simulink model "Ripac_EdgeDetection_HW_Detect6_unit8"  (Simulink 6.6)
settings: Solver=FixedStepDiscrete  SolverMode=SingleTasking  StartTime=0.0  StopTime=row  RelTol=1e-3
PreLoadFcn:
  | [r,g,b]=Ripac_img_start('image.jpg');
  | 
  | col=r.signals.dimensions;
  | row=size(r.signals.values,1);
  | 
  | kernel = [-1 0 1; -2 0 2; -1 0 1];
  | gain_frac=0;
InitFcn:
  | %[r,g,b]=Ripac_img_start('image.jpg');
  | 
  | %col=r.signals.dimensions;
  | %row=size(r.signals.values,1);
  | 
  | %kernel = [-1 0 1; -2 0 2; -1 0 1];
  | 
  | gain_frac=0;
StopFcn:
  | obr_out=Ripac_img_stop(hrana,col);
  | obr=int16((double(obr_out)).^(1/2));
  | figure, image(obr); colormap('gray'), title('Final Edge Detected Image')
  | 
  | output_struct=hrana8;
  | obr2_out=reshape(output_struct.signals.values(1:end-1),col+2,prod(size(output_struct.signals.values(1:end-1)))/(col+2))';
  | obr2=int16(obr2_out.^(1/2));
  | figure,image(obr2); colormap('gray'), title('HW Edge Detected Image')
libraries: syndsplibv9 x42, simulink x8, dspbuff3 x1

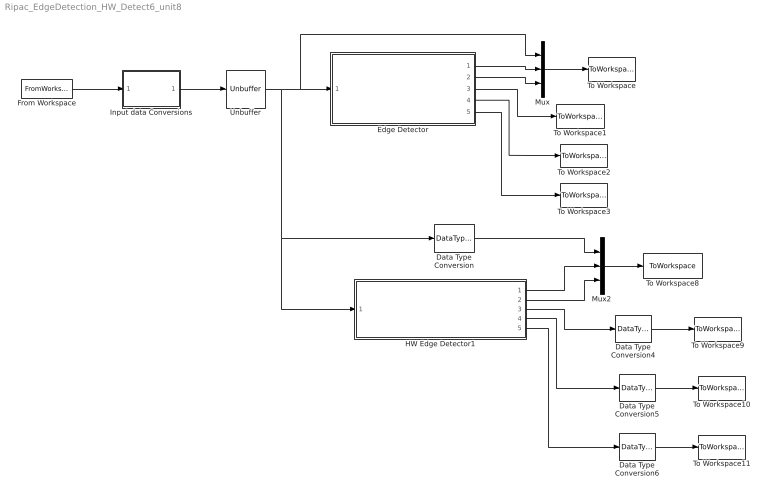
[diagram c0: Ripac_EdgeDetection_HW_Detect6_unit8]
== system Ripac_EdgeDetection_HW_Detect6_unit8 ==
  Data Type Conversion : DataTypeConversion  OutDataTypeMode=int16
  Data Type Conversion4 : DataTypeConversion  OutDataTypeMode=double  RndMeth=Nearest
  Data Type Conversion5 : DataTypeConversion  OutDataTypeMode=int32  RndMeth=Nearest
  Data Type Conversion6 : DataTypeConversion  OutDataTypeMode=int32  RndMeth=Nearest
  Edge Detector : Subsystem
  From Workspace : FromWorkspace  VariableName=r  SampleTime=0  Interpolate=off  OutputAfterFinalValue=Setting to zero
  HW Edge Detector1 : Subsystem
  Input data Conversions : Subsystem
  Mux : Mux  Inputs=3
  Mux2 : Mux  Inputs=3
  To Workspace : ToWorkspace  VariableName=simout  SampleTime=-1  SaveFormat=Structure With Time
  To Workspace1 : ToWorkspace  VariableName=hrana  SampleTime=-1  SaveFormat=Structure With Time
  To Workspace10 : ToWorkspace  VariableName=hrana6  SampleTime=-1  SaveFormat=Structure With Time
  To Workspace11 : ToWorkspace  VariableName=hrana7  SampleTime=-1  SaveFormat=Structure With Time
  To Workspace2 : ToWorkspace  VariableName=hrana1  SampleTime=-1  SaveFormat=Structure With Time
  To Workspace3 : ToWorkspace  VariableName=hrana2  SampleTime=-1  SaveFormat=Structure With Time
  To Workspace8 : ToWorkspace  VariableName=simout_HW1  SampleTime=-1  SaveFormat=Structure With Time
  To Workspace9 : ToWorkspace  VariableName=hrana8  SampleTime=-1  SaveFormat=Structure With Time
  Unbuffer : dspbuff3/Unbuffer  ic=0
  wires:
  From Workspace/1 -> Input data Conversions/1(In)
  Unbuffer/1 -> Mux/1, Edge Detector/1(Row Input), HW Edge Detector1/1(In1), Data Type Conversion/1
  Input data Conversions/1(Out) -> Unbuffer/1
  Edge Detector/3(Detector Out) -> To Workspace1/1
  Mux/1 -> To Workspace/1
  Edge Detector/1(Delay Line Out 1) -> Mux/2
  Edge Detector/2(Delay Line Out 2) -> Mux/3
  Edge Detector/4(Detector Out1) -> To Workspace2/1
  Edge Detector/5(Detector Out2) -> To Workspace3/1
  HW Edge Detector1/1(Delay Line 1) -> Mux2/2
  HW Edge Detector1/2("Delay Line 2 ") -> Mux2/3
  Mux2/1 -> To Workspace8/1
  Data Type Conversion4/1 -> To Workspace9/1
  Data Type Conversion5/1 -> To Workspace10/1
  HW Edge Detector1/3(Edge2) -> Data Type Conversion4/1
  HW Edge Detector1/4(Edge) -> Data Type Conversion5/1
  HW Edge Detector1/5(Edge1) -> Data Type Conversion6/1
  Data Type Conversion6/1 -> To Workspace11/1
  Data Type Conversion/1 -> Mux2/1

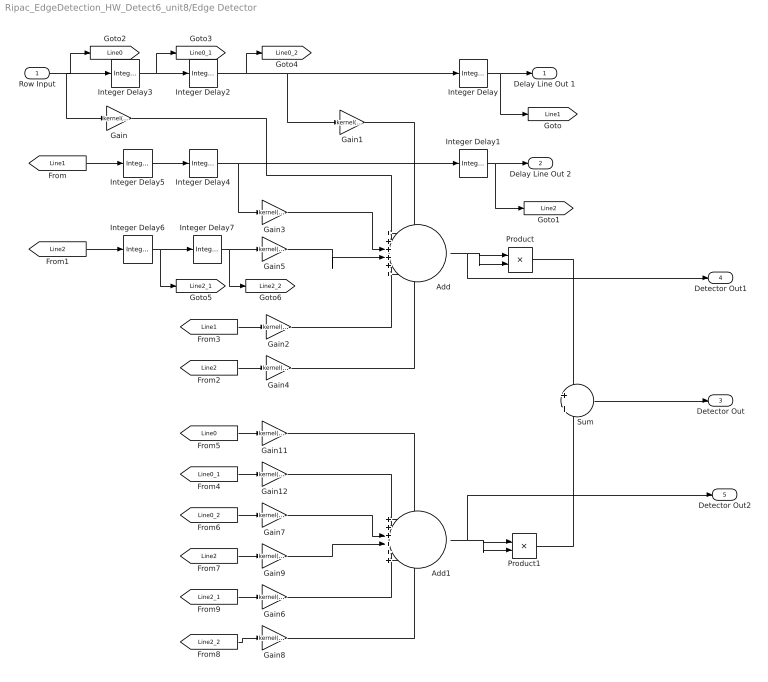
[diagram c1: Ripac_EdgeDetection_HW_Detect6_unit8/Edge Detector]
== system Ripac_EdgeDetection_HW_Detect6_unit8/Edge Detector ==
  Row Input : Inport  OutDataType=fixdt(1,16,0)  OutScaling=[]
  Add : Sum  Inputs=++++++  OutScaling=2^-10
  Add1 : Sum  Inputs=++++++  OutScaling=2^-10
  Gain : Gain  Gain=kernel(1,1)
  Gain1 : Gain  Gain=kernel(1,3)
  Gain11 : Gain  Gain=kernel(1,1)
  Gain12 : Gain  Gain=kernel(2,1)
  Gain2 : Gain  Gain=kernel(2,1)
  Gain3 : Gain  Gain=kernel(2,3)
  Gain4 : Gain  Gain=kernel(3,1)
  Gain5 : Gain  Gain=kernel(3,3)
  Gain6 : Gain  Gain=kernel(2,3)
  Gain7 : Gain  Gain=kernel(3,1)
  Gain8 : Gain  Gain=kernel(3,3)
  Gain9 : Gain  Gain=kernel(1,3)
  Integer Delay : simulink/Discrete/Integer Delay  vinit=0.0  samptime=-1  NumDelays=col
  Integer Delay1 : simulink/Discrete/Integer Delay  vinit=0.0  samptime=-1  NumDelays=col
  Integer Delay{2..7} (6 alike) : simulink/Discrete/Integer Delay  vinit=0.0  samptime=-1  NumDelays=1
  Product : Product  OutDataTypeMode=double
  Product1 : Product  OutDataTypeMode=double
  Sum : Sum  Inputs=+|+
  Delay Line Out 1 : Outport  OutDataType=fixdt(1,16,0)  OutScaling=[]
  Delay Line Out 2 : Outport  Port=2  OutDataType=fixdt(1,16,0)  OutScaling=[]
  Detector Out : Outport  Port=3  OutDataType=fixdt(1,16,0)  OutScaling=[]
  Detector Out1 : Outport  Port=4  OutDataType=fixdt(1,16,0)  OutScaling=[]
  Detector Out2 : Outport  Port=5  OutDataType=fixdt(1,16,0)  OutScaling=[]
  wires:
  Integer Delay/1 -> Delay Line Out 1/1, [Line1]
  Integer Delay3/1 -> [Line0_1], Integer Delay2/1
  Integer Delay2/1 -> Integer Delay/1, Gain1/1, [Line0_2]
  Integer Delay5/1 -> Integer Delay4/1
  Integer Delay4/1 -> Gain3/1, Integer Delay1/1
  Integer Delay6/1 -> [Line2_1], Integer Delay7/1
  Integer Delay7/1 -> Gain5/1, [Line2_2]
  Integer Delay1/1 -> Delay Line Out 2/1, [Line2]
  Gain1/1 -> Add/1
  Gain4/1 -> Add/6
  Row Input/1 -> Gain/1, [Line0], Integer Delay3/1
  [Line1] -> Integer Delay5/1
  [Line2] -> Integer Delay6/1
  [Line2] -> Gain4/1
  [Line1] -> Gain2/1
  Gain/1 -> Add/2
  Gain3/1 -> Add/3
  Gain5/1 -> Add/4
  Gain2/1 -> Add/5
  Gain11/1 -> Add1/1
  Gain8/1 -> Add1/6
  Add1/1 -> Product1/1, Product1/2, Detector Out2/1
  Gain12/1 -> Add1/2
  Gain7/1 -> Add1/3
  Gain9/1 -> Add1/4
  Gain6/1 -> Add1/5
  [Line0] -> Gain11/1
  [Line0_2] -> Gain7/1
  [Line0_1] -> Gain12/1
  [Line2] -> Gain9/1
  [Line2_1] -> Gain6/1
  [Line2_2] -> Gain8/1
  Add/1 -> Product/1, Product/2, Detector Out1/1
  Product/1 -> Sum/1
  Product1/1 -> Sum/2
  Sum/1 -> Detector Out/1

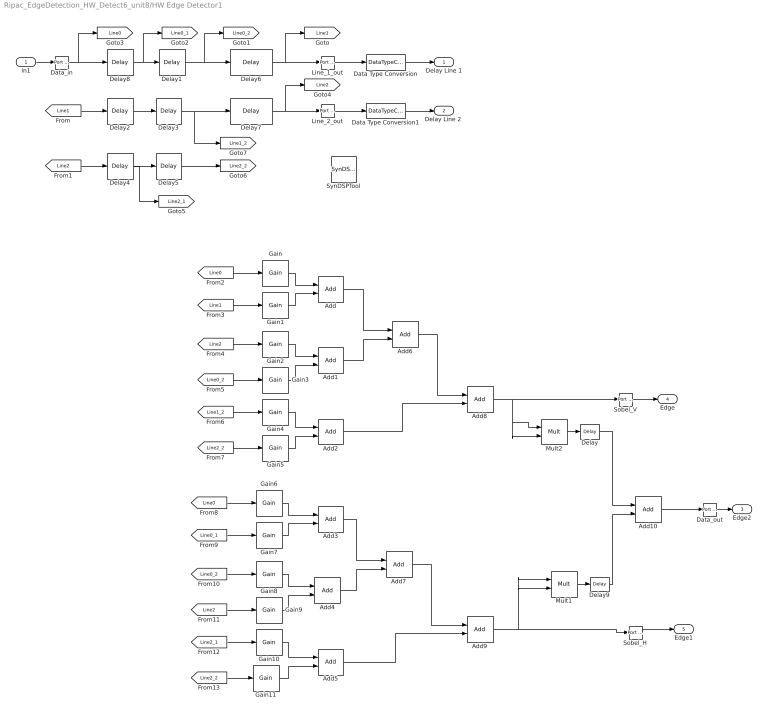
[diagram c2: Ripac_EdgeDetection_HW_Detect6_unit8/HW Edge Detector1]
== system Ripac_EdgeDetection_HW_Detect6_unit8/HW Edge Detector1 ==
  In1 : Inport  OutDataType=fixdt(1,16,0)  OutScaling=[]
  Add{,1..10} (11 alike) : syndsplibv9/Math Functions/Add  syn_add_opr=++  syn_out_f=Automatic  syn_out_wl=16  syn_out_fl=8  syn_out_dt=signed  syn_out_sat=off  syn_out_rnd=Floor (Truncate)  synBlockType=primitive  synLatency=0  synBlockId=96
  Data Type Conversion : DataTypeConversion  OutDataTypeMode=int16
  Data Type Conversion1 : DataTypeConversion  OutDataTypeMode=int16
  Data_in : syndsplibv9/Ports & Subsystems/Port In  syn_out_wl=8  syn_out_fl=0  syn_out_dt=unsigned  syn_out_st=-1  syn_capture=off  syn_register=off  syn_out_sat=off  syn_out_rnd=on  synBlockType=port  synLatency=0  synBlockId=0
  Data_out : syndsplibv9/Ports & Subsystems/Port Out  syn_capture=on  syn_register=off  synBlockType=port  synLatency=0  synBlockId=1
  Delay : syndsplibv9/Memories/Delay  syn_delay_val=3  synBlockType=primitive  synLatency=3  synBlockId=104
  Delay{1..5,8} (6 alike) : syndsplibv9/Memories/Delay  syn_delay_val=1  synBlockType=primitive  synLatency=1  synBlockId=104
  Delay6 : syndsplibv9/Memories/Delay  syn_delay_val=col  synBlockType=primitive  synLatency=1024  synBlockId=104
  Delay7 : syndsplibv9/Memories/Delay  syn_delay_val=col  synBlockType=primitive  synLatency=1024  synBlockId=104
  Delay9 : syndsplibv9/Memories/Delay  syn_delay_val=3  synBlockType=primitive  synLatency=3  synBlockId=104
  Gain : syndsplibv9/Math Functions/Gain  syn_gain_val=kernel(1,1)  syn_gain_fl=gain_frac  syn_gain_dt=signed  syn_gain_rnd=on  syn_out_f=Full Precision  syn_out_wl=16  syn_out_fl=8  syn_out_dt=signed  syn_out_sat=off  syn_out_rnd=Floor (Truncate)  synBlockType=primitive  synLatency=0  synBlockId=3  syn_opr_mode=0
  Gain1 : syndsplibv9/Math Functions/Gain  syn_gain_val=kernel(2,1)  syn_gain_fl=gain_frac  syn_gain_dt=signed  syn_gain_rnd=on  syn_out_f=Full Precision  syn_out_wl=16  syn_out_fl=8  syn_out_dt=signed  syn_out_sat=off  syn_out_rnd=Floor (Truncate)  synBlockType=primitive  synLatency=0  synBlockId=3  syn_opr_mode=0
  Gain10 : syndsplibv9/Math Functions/Gain  syn_gain_val=kernel(2,3)  syn_gain_fl=gain_frac  syn_gain_dt=signed  syn_gain_rnd=on  syn_out_f=Full Precision  syn_out_wl=16  syn_out_fl=8  syn_out_dt=signed  syn_out_sat=off  syn_out_rnd=Floor (Truncate)  synBlockType=primitive  synLatency=0  synBlockId=3  syn_opr_mode=0
  Gain11 : syndsplibv9/Math Functions/Gain  syn_gain_val=kernel(3,3)  syn_gain_fl=gain_frac  syn_gain_dt=signed  syn_gain_rnd=on  syn_out_f=Full Precision  syn_out_wl=16  syn_out_fl=8  syn_out_dt=signed  syn_out_sat=off  syn_out_rnd=Floor (Truncate)  synBlockType=primitive  synLatency=0  synBlockId=3  syn_opr_mode=0
  Gain2 : syndsplibv9/Math Functions/Gain  syn_gain_val=kernel(3,1)  syn_gain_fl=gain_frac  syn_gain_dt=signed  syn_gain_rnd=on  syn_out_f=Full Precision  syn_out_wl=16  syn_out_fl=8  syn_out_dt=signed  syn_out_sat=off  syn_out_rnd=Floor (Truncate)  synBlockType=primitive  synLatency=0  synBlockId=3  syn_opr_mode=0
  Gain3 : syndsplibv9/Math Functions/Gain  syn_gain_val=kernel(1,3)  syn_gain_fl=gain_frac  syn_gain_dt=signed  syn_gain_rnd=on  syn_out_f=Full Precision  syn_out_wl=16  syn_out_fl=8  syn_out_dt=signed  syn_out_sat=off  syn_out_rnd=Floor (Truncate)  synBlockType=primitive  synLatency=0  synBlockId=3  syn_opr_mode=0
  Gain4 : syndsplibv9/Math Functions/Gain  syn_gain_val=kernel(2,3)  syn_gain_fl=gain_frac  syn_gain_dt=signed  syn_gain_rnd=on  syn_out_f=Full Precision  syn_out_wl=16  syn_out_fl=8  syn_out_dt=signed  syn_out_sat=off  syn_out_rnd=Floor (Truncate)  synBlockType=primitive  synLatency=0  synBlockId=3  syn_opr_mode=0
  Gain5 : syndsplibv9/Math Functions/Gain  syn_gain_val=kernel(3,3)  syn_gain_fl=gain_frac  syn_gain_dt=signed  syn_gain_rnd=on  syn_out_f=Full Precision  syn_out_wl=16  syn_out_fl=8  syn_out_dt=signed  syn_out_sat=off  syn_out_rnd=Floor (Truncate)  synBlockType=primitive  synLatency=0  synBlockId=3  syn_opr_mode=0
  Gain6 : syndsplibv9/Math Functions/Gain  syn_gain_val=kernel(1,1)  syn_gain_fl=gain_frac  syn_gain_dt=signed  syn_gain_rnd=on  syn_out_f=Full Precision  syn_out_wl=16  syn_out_fl=8  syn_out_dt=signed  syn_out_sat=off  syn_out_rnd=Floor (Truncate)  synBlockType=primitive  synLatency=0  synBlockId=3  syn_opr_mode=0
  Gain7 : syndsplibv9/Math Functions/Gain  syn_gain_val=kernel(2,1)  syn_gain_fl=gain_frac  syn_gain_dt=signed  syn_gain_rnd=on  syn_out_f=Full Precision  syn_out_wl=16  syn_out_fl=8  syn_out_dt=signed  syn_out_sat=off  syn_out_rnd=Floor (Truncate)  synBlockType=primitive  synLatency=0  synBlockId=3  syn_opr_mode=0
  Gain8 : syndsplibv9/Math Functions/Gain  syn_gain_val=kernel(3,1)  syn_gain_fl=gain_frac  syn_gain_dt=signed  syn_gain_rnd=on  syn_out_f=Full Precision  syn_out_wl=16  syn_out_fl=8  syn_out_dt=signed  syn_out_sat=off  syn_out_rnd=Floor (Truncate)  synBlockType=primitive  synLatency=0  synBlockId=3  syn_opr_mode=0
  Gain9 : syndsplibv9/Math Functions/Gain  syn_gain_val=kernel(1,3)  syn_gain_fl=gain_frac  syn_gain_dt=signed  syn_gain_rnd=on  syn_out_f=Full Precision  syn_out_wl=16  syn_out_fl=8  syn_out_dt=signed  syn_out_sat=off  syn_out_rnd=Floor (Truncate)  synBlockType=primitive  synLatency=0  synBlockId=3  syn_opr_mode=0
  Line_1_out : syndsplibv9/Ports & Subsystems/Port Out  syn_capture=on  syn_register=off  synBlockType=port  synLatency=0  synBlockId=1
  Line_2_out : syndsplibv9/Ports & Subsystems/Port Out  syn_capture=on  syn_register=off  synBlockType=port  synLatency=0  synBlockId=1
  Mult1 : syndsplibv9/Math Functions/Mult  syn_out_f=Full Precision  syn_out_wl=16  syn_out_fl=8  syn_out_dt=signed  syn_out_sat=off  syn_out_rnd=Floor (Truncate)  synBlockType=primitive  synLatency=0  synBlockId=3  syn_opr_mode=1
  Mult2 : syndsplibv9/Math Functions/Mult  syn_out_f=Full Precision  syn_out_wl=16  syn_out_fl=8  syn_out_dt=signed  syn_out_sat=off  syn_out_rnd=Floor (Truncate)  synBlockType=primitive  synLatency=0  synBlockId=3  syn_opr_mode=1
  Sobel_H : syndsplibv9/Ports & Subsystems/Port Out  syn_capture=on  syn_register=off  synBlockType=port  synLatency=0  synBlockId=1
  Sobel_V : syndsplibv9/Ports & Subsystems/Port Out  syn_capture=on  syn_register=off  synBlockType=port  synLatency=0  synBlockId=1
  SynDSPTool : syndsplibv9/SynDSPTool  SystemSampleTime=-1  synBlockType=tool  syn_dsp_mode=FPGA
  Delay Line 1 : Outport  OutDataType=fixdt(1,16,0)  OutScaling=[]
  "Delay Line 2 " : Outport  Port=2  OutDataType=fixdt(1,16,0)  OutScaling=[]
  Edge2 : Outport  Port=3  OutDataType=fixdt(1,16,0)  OutScaling=[]
  Edge : Outport  Port=4  OutDataType=fixdt(1,16,0)  OutScaling=[]
  Edge1 : Outport  Port=5  OutDataType=fixdt(1,16,0)  OutScaling=[]
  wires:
  Data_out/1 -> Edge2/1
  Add10/1 -> Data_out/1
  Mult1/1 -> Delay9/1
  Mult2/1 -> Delay/1
  Sobel_H/1 -> Edge1/1
  Add9/1 -> Mult1/1, Mult1/2, Sobel_H/1
  Add5/1 -> Add9/2
  Add7/1 -> Add9/1
  Add4/1 -> Add7/2
  Add3/1 -> Add7/1
  Gain11/1 -> Add5/2
  Gain10/1 -> Add5/1
  Gain9/1 -> Add4/2
  Gain8/1 -> Add4/1
  Gain7/1 -> Add3/2
  Gain6/1 -> Add3/1
  [Line2_2] -> Gain11/1
  [Line2_1] -> Gain10/1
  [Line2] -> Gain9/1
  [Line0_2] -> Gain8/1
  [Line0_1] -> Gain7/1
  [Line0] -> Gain6/1
  Sobel_V/1 -> Edge/1
  Add8/1 -> Mult2/2, Mult2/1, Sobel_V/1
  Add2/1 -> Add8/2
  Add6/1 -> Add8/1
  Add1/1 -> Add6/2
  Add/1 -> Add6/1
  Gain5/1 -> Add2/2
  Gain4/1 -> Add2/1
  Gain3/1 -> Add1/2
  Gain2/1 -> Add1/1
  Gain1/1 -> Add/2
  Gain/1 -> Add/1
  [Line2_2] -> Gain5/1
  [Line1_2] -> Gain4/1
  [Line0_2] -> Gain3/1
  [Line2] -> Gain2/1
  [Line1] -> Gain1/1
  [Line0] -> Gain/1
  Delay5/1 -> [Line2_2]
  Delay7/1 -> [Line2], Line_2_out/1
  [Line2] -> Delay4/1
  [Line1] -> Delay2/1
  Delay6/1 -> [Line1], Line_1_out/1
  Delay4/1 -> [Line2_1], Delay5/1
  Delay3/1 -> [Line1_2], Delay7/1
  Delay2/1 -> Delay3/1
  Delay1/1 -> [Line0_2], Delay6/1
  Delay8/1 -> [Line0_1], Delay1/1
  Data Type Conversion1/1 -> "Delay Line 2 "/1
  Data Type Conversion/1 -> Delay Line 1/1
  Line_2_out/1 -> Data Type Conversion1/1
  Line_1_out/1 -> Data Type Conversion/1
  In1/1 -> Data_in/1
  Data_in/1 -> [Line0], Delay8/1
  Delay/1 -> Add10/1
  Delay9/1 -> Add10/2

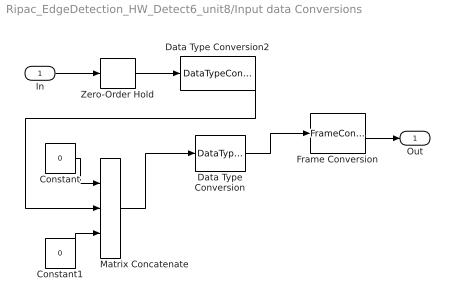
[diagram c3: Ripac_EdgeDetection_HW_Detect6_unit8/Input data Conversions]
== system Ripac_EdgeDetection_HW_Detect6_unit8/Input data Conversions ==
  In : Inport  OutDataType=fixdt(1,16,0)  OutScaling=[]
  Constant : Constant  Value=0
  Constant1 : Constant  Value=0
  Data Type Conversion : DataTypeConversion  OutDataTypeMode=Specify via dialog  OutDataType=fixdt(1,9,0)  OutScaling=[]
  Data Type Conversion2 : DataTypeConversion  OutDataTypeMode=double
  Frame Conversion : FrameConversion
  Matrix Concatenate : Concatenate  NumInputs=3  Mode=Vector  ConcatenateDimension=2
  Zero-Order Hold : ZeroOrderHold
  Out : Outport  OutDataType=fixdt(1,16,0)  OutScaling=[]
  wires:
  Zero-Order Hold/1 -> Data Type Conversion2/1
  Data Type Conversion/1 -> Frame Conversion/1
  Matrix Concatenate/1 -> Data Type Conversion/1
  Constant/1 -> Matrix Concatenate/1
  Constant1/1 -> Matrix Concatenate/3
  Data Type Conversion2/1 -> Matrix Concatenate/2
  In/1 -> Zero-Order Hold/1
  Frame Conversion/1 -> Out/1
